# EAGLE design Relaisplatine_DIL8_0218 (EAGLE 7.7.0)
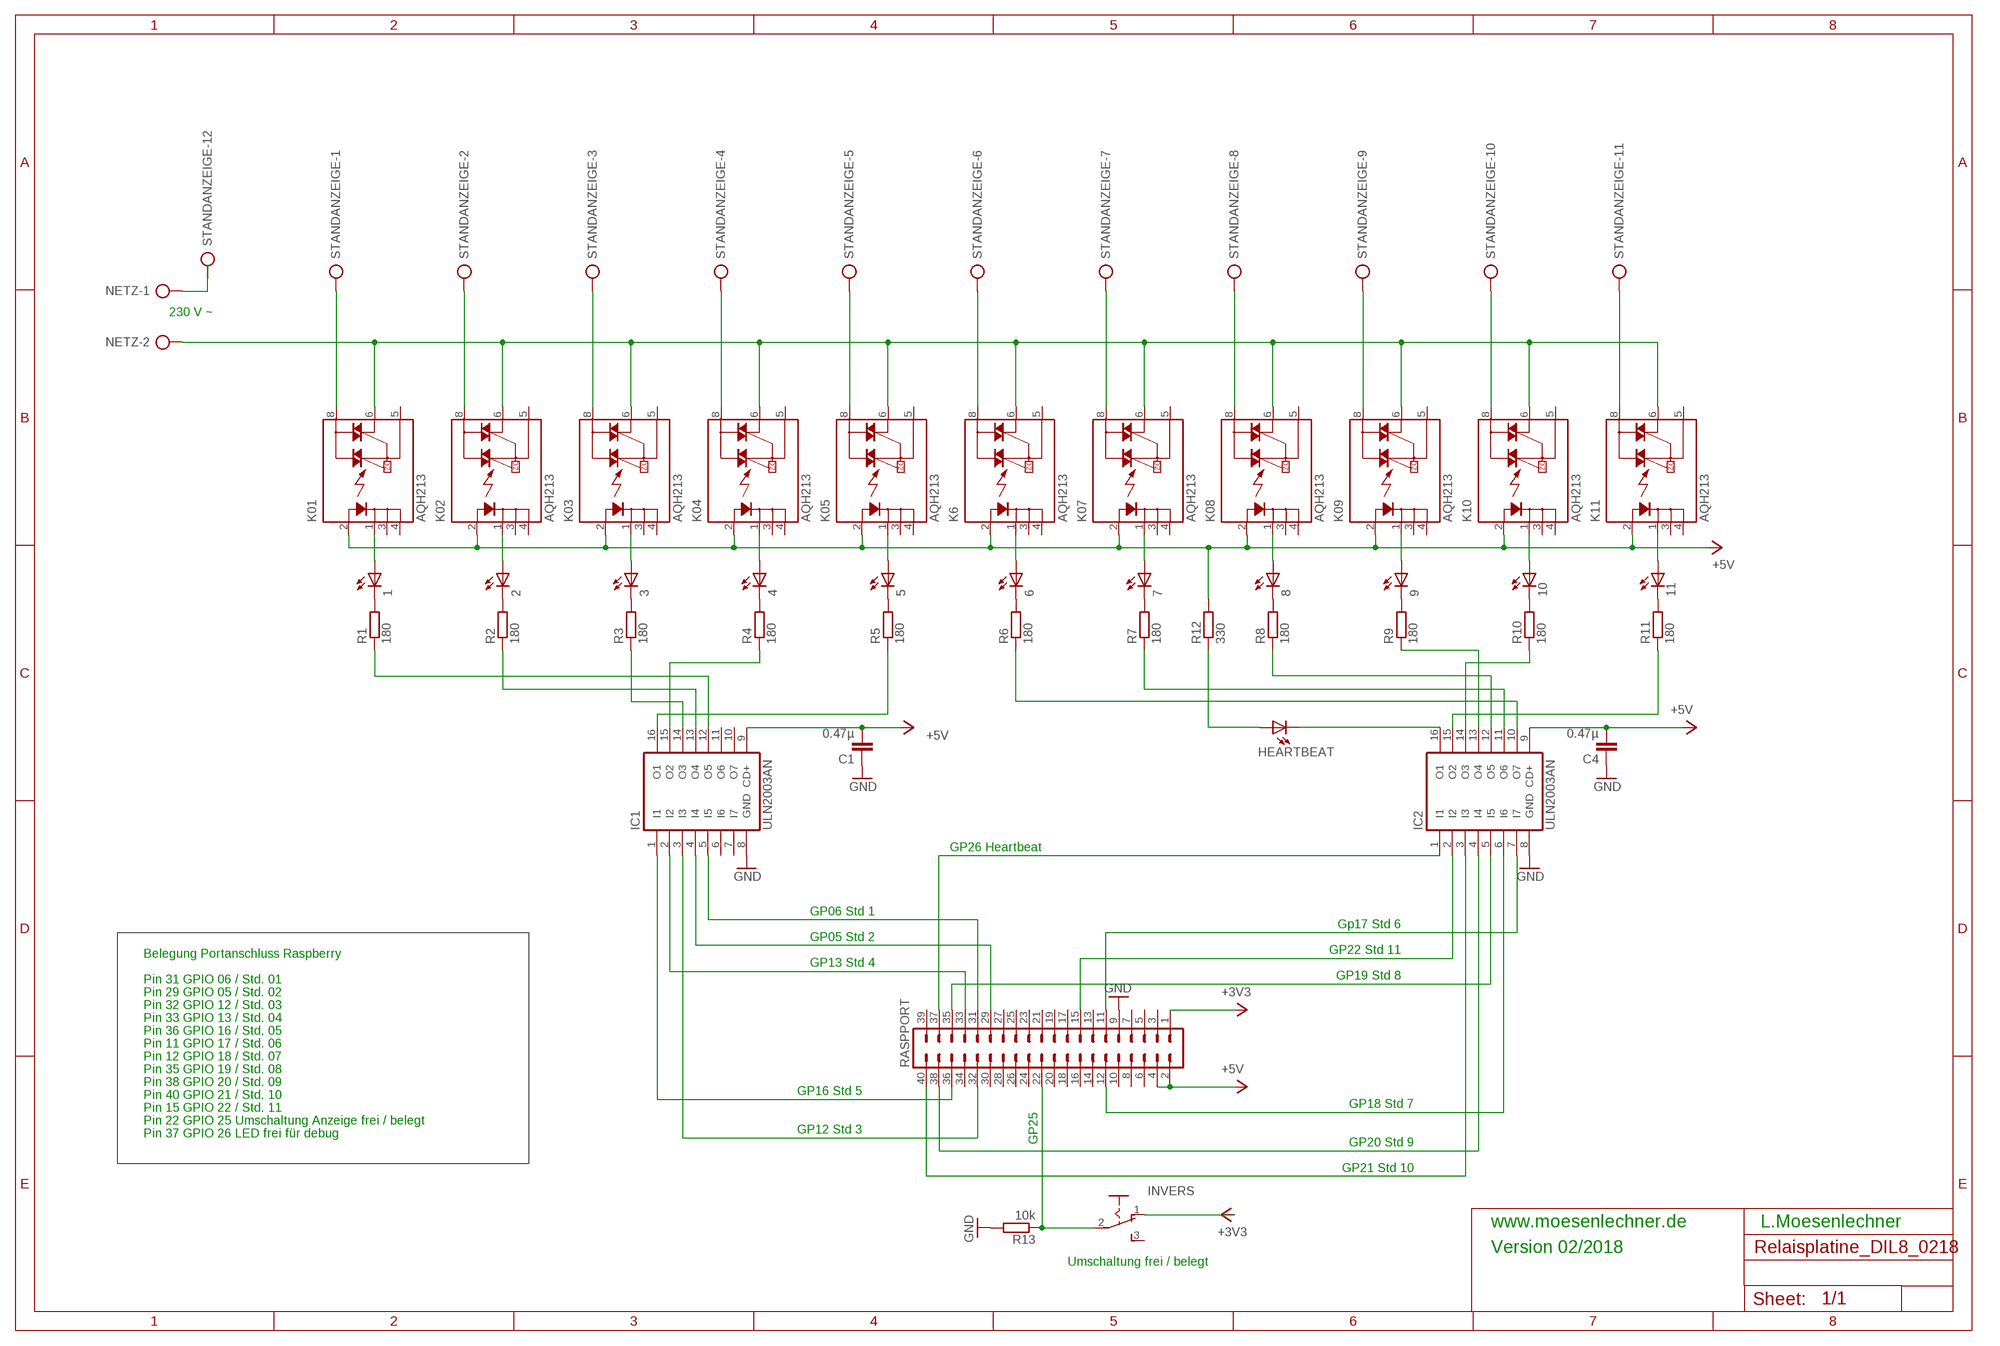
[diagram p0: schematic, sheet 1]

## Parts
1  LS_T679-D2E2-1  [PLCC2]
2  LS_T679-D2E2-1  [PLCC2]
3  LS_T679-D2E2-1  [PLCC2]
4  LS_T679-D2E2-1  [PLCC2]
5  LS_T679-D2E2-1  [PLCC2]
6  LS_T679-D2E2-1  [PLCC2]
7  LS_T679-D2E2-1  [PLCC2]
8  LS_T679-D2E2-1  [PLCC2]
9  LS_T679-D2E2-1  [PLCC2]
10  LS_T679-D2E2-1  [PLCC2]
11  LS_T679-D2E2-1  [PLCC2]
C1  0.47µ  C-EUC1206K  [C1206K]
C4  0.47µ  C-EUC1206K  [C1206K]
HEARTBEAT  LS_T679-D2E2-1  [PLCC2]
IC1  ULN2003AN  [DIL16]
IC2  ULN2003AN  [DIL16]
INVERS  M251  [M251]
K01  AQH213  [DIL07]
K02  AQH213  [DIL07]
K03  AQH213  [DIL07]
K04  AQH213  [DIL07]
K05  AQH213  [DIL07]
K6  AQH213  [DIL07]
K07  AQH213  [DIL07]
K08  AQH213  [DIL07]
K09  AQH213  [DIL07]
K10  AQH213  [DIL07]
K11  AQH213  [DIL07]
NETZ  AK500/2-H  [AK500/2-H]
R1  180  R-EU_R1206W  [R1206W]
R2  180  R-EU_R1206W  [R1206W]
R3  180  R-EU_R1206W  [R1206W]
R4  180  R-EU_R1206W  [R1206W]
R5  180  R-EU_R1206W  [R1206W]
R6  180  R-EU_R1206W  [R1206W]
R7  180  R-EU_R1206W  [R1206W]
R8  180  R-EU_R1206W  [R1206W]
R9  180  R-EU_R1206W  [R1206W]
R10  180  R-EU_R1206W  [R1206W]
R11  180  R-EU_R1206W  [R1206W]
R12  330  R-EU_R1206W  [R1206W]
R13  10k  R-EU_R1206W  [R1206W]
RASPPORT  MA20-2  [MA20-2]
STANDANZEIGE  AK500/12-H  [AK500/12-H]

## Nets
+3V3: INVERS.1(O) RASPPORT.1
+5V: C1.2 C4.2 IC1.9(CD+) IC2.9(CD+) K01.2(A) K02.2(A) K03.2(A) K04.2(A) K05.2(A) K6.2(A) K07.2(A) K08.2(A) K09.2(A) K10.2(A) K11.2(A) R12.2 RASPPORT.2 RASPPORT.4
GND: C1.1 C4.1 IC1.8(GND) IC2.8(GND) R13.2 RASPPORT.9
N$1: K01.8(DS1) STANDANZEIGE.1
N$2: K02.8(DS1) STANDANZEIGE.2
N$3: K03.8(DS1) STANDANZEIGE.3
N$4: K04.8(DS1) STANDANZEIGE.4
N$5: K05.8(DS1) STANDANZEIGE.5
N$6: K6.8(DS1) STANDANZEIGE.6
N$7: K07.8(DS1) STANDANZEIGE.7
N$8: K08.8(DS1) STANDANZEIGE.8
N$9: K09.8(DS1) STANDANZEIGE.9
N$10: K10.8(DS1) STANDANZEIGE.10
N$11: K11.8(DS1) STANDANZEIGE.11
N$12: K01.6(DS3) K02.6(DS3) K03.6(DS3) K04.6(DS3) K05.6(DS3) K6.6(DS3) K07.6(DS3) K08.6(DS3) K09.6(DS3) K10.6(DS3) K11.6(DS3) NETZ.2
N$13: 9.C R9.2
N$14: IC1.16(O1) R5.1
N$15: IC1.5(I5) RASPPORT.31
N$16: 10.C R10.2
N$17: 2.C R2.2
N$18: IC1.13(O4) R2.1
N$19: 11.C R11.2
N$20: IC2.10(O7) R6.1
N$21: IC2.11(O6) R7.1
N$22: 3.C R3.2
N$23: 4.C R4.2
N$24: 5.C R5.2
N$25: IC2.12(O5) R8.1
N$26: IC2.4(I4) RASPPORT.38
N$27: IC2.13(O4) R9.1
N$28: IC2.15(O2) R11.1
N$29: IC2.14(O3) R10.1
N$30: IC2.7(I7) RASPPORT.11
N$31: IC1.14(O3) R3.1
N$32: IC1.15(O2) R4.1
N$33: IC1.12(O5) R1.1
N$35: IC2.6(I6) RASPPORT.12
N$36: IC2.5(I5) RASPPORT.35
N$37: IC2.3(I3) RASPPORT.40
N$38: 1.C R1.2
N$39: 6.C R6.2
N$40: 7.C R7.2
N$41: 8.C R8.2
N$42: IC2.2(I2) RASPPORT.15
N$43: NETZ.1 STANDANZEIGE.12
N$44: 1.A K01.1(K)
N$45: 2.A K02.1(K)
N$46: 3.A K03.1(K)
N$47: 4.A K04.1(K)
N$48: 5.A K05.1(K)
N$49: 6.A K6.1(K)
N$50: IC1.1(I1) RASPPORT.36
N$51: IC1.3(I3) RASPPORT.32
N$52: IC1.2(I2) RASPPORT.33
N$53: 7.A K07.1(K)
N$54: 8.A K08.1(K)
N$55: 9.A K09.1(K)
N$56: 10.A K10.1(K)
N$57: 11.A K11.1(K)
N$58: HEARTBEAT.C IC2.16(O1)
N$59: HEARTBEAT.A R12.1
N$60: INVERS.2(P) R13.1 RASPPORT.22
N$61: IC2.1(I1) RASPPORT.37
N$62: IC1.4(I4) RASPPORT.29
Unconnected: IC1.6(I6) IC1.7(I7) IC1.10(O7) IC1.11(O6) INVERS.3(S) K01.3(K1) K01.4(K2) K01.5(DS2) K02.3(K1) K02.4(K2) K02.5(DS2) K03.3(K1) K03.4(K2) K03.5(DS2) K04.3(K1) K04.4(K2) K04.5(DS2) K05.3(K1) K05.4(K2) K05.5(DS2) K6.3(K1) K6.4(K2) K6.5(DS2) K07.3(K1) K07.4(K2) K07.5(DS2) K08.3(K1) K08.4(K2) K08.5(DS2) K09.3(K1) K09.4(K2) K09.5(DS2) K10.3(K1) K10.4(K2) K10.5(DS2) K11.3(K1) K11.4(K2) K11.5(DS2) RASPPORT.3 RASPPORT.5 RASPPORT.6 RASPPORT.7 RASPPORT.8 RASPPORT.10 RASPPORT.13 RASPPORT.14 RASPPORT.16 RASPPORT.17 RASPPORT.18 RASPPORT.19 RASPPORT.20 RASPPORT.21 RASPPORT.23 RASPPORT.24 RASPPORT.25 RASPPORT.26 RASPPORT.27 RASPPORT.28 RASPPORT.30 RASPPORT.34 RASPPORT.39

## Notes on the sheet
- 230 V ~
- GP26 Heartbeat
- GP06 Std 1
- Gp17 Std 6
- GP05 Std 2
- GP22 Std 11
- Belegung Portanschluss Raspberry | GP13 Std 4
- GP19 Std 8
- Pin 31 GPIO 06 / Std. 01
- Pin 29 GPIO 05 / Std. 02
- Pin 32 GPIO 12 / Std. 03
- Pin 33 GPIO 13 / Std. 04
- Pin 36 GPIO 16 / Std. 05
- Pin 11 GPIO 17 / Std. 06
- Pin 12 GPIO 18 / Std. 07
- Pin 35 GPIO 19 / Std. 08
- Pin 38 GPIO 20 / Std. 09 | GP16 Std 5
- Pin 40 GPIO 21 / Std. 10 | GP18 Std 7
- Pin 15 GPIO 22 / Std. 11 | GP25
- Pin 22 GPIO 25 Umschaltung Anzeige frei / belegt | GP12 Std 3
- Pin 37 GPIO 26 LED frei für debug | GP20 Std 9
- GP21 Std 10
- www.moesenlechner.de | L.Moesenlechner
- Version 02/2018
- Umschaltung frei / belegt

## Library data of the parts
1-11 HEARTBEAT = led:*_T679-?-1: LC TOPLED® Low Current LED; COLOR: super-red
C1 C4 = rcl:C-EU: CAPACITOR, European symbol
IC1 IC2 = uln-udn:ULN2003A: DRIVER ARRAY
INVERS = switch:M251: SLIDING SWITCH Mors, distributor Buerklin, 11G702
K01-K05 K6 K07-K09 K10 K11 = relay:AQH*213: SOLID STATE RELAY NAiS Source: http://www.mew-europe.com/.. en_ds_61613_0000.pdf; OC_FARNELL: unknown; OC_NEWARK: unknown
NETZ = con-ptr500:AK500/2-H: CONNECTOR; OC_FARNELL: unknown; OC_NEWARK: unknown
R1-R13 = rcl:R-EU_: RESISTOR, European symbol
RASPPORT = con-lstb:MA20-2: PIN HEADER; OC_FARNELL: unknown; OC_NEWARK: unknown
STANDANZEIGE = con-ptr500:AK500/12-H: CONNECTOR Aug. 2004 / PTR Meßtechnik: Die Bezeichnung der Serie AK505 wurde geändert. Es handelt sich hierbei um AK500 in horizontaler Ausführung.; OC_FARNELL: unknown; OC_NEWARK: unknown

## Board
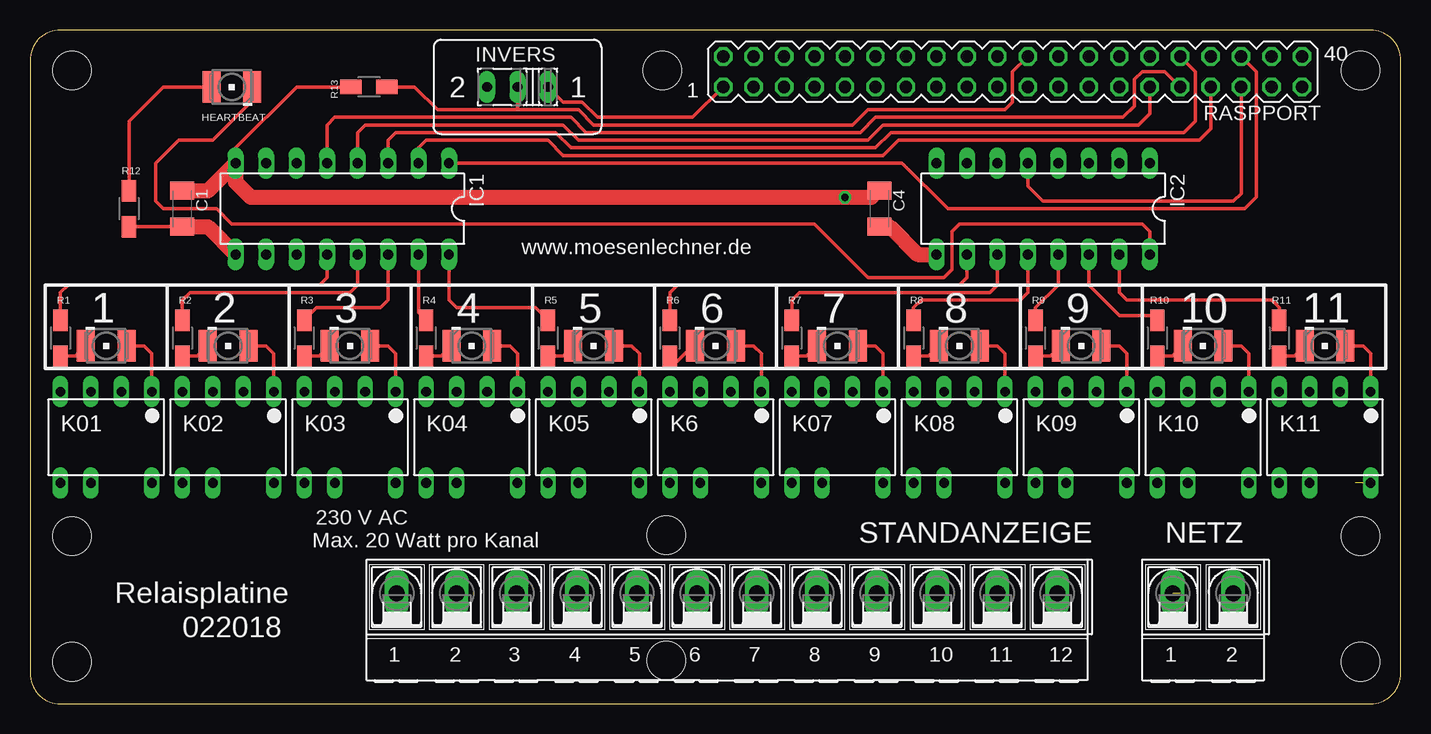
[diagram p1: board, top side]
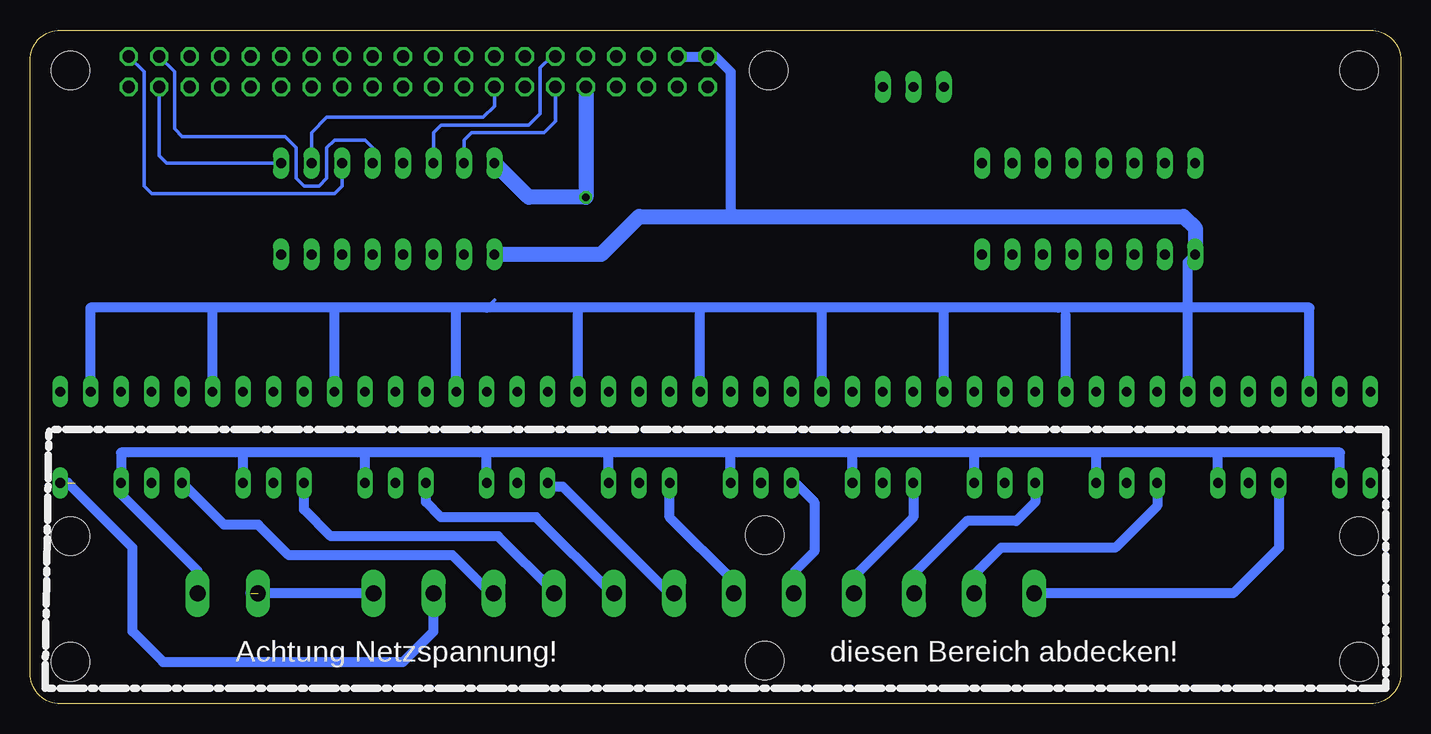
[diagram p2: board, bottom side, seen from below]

Size 114.28 x 56.19 mm. Coordinates in mm from the lower left corner, seen from the top.
Outline: 0,53.65 0,2.54 arc90 2.54,0 111.74,0 arc90 114.28,2.54 114.28,53.65 arc90 111.74,56.19 2.54,56.19 arc90 0,53.65
Copper layers (1*16): Top 0.035mm / dielectric 1.5mm / Bottom 0.035mm
Design rules "default": minimum track width 10mil, minimum drill 24mil, track to track 8mil, track to pad 8mil, pad to pad 8mil, via to via 8mil, smd to smd 8mil, copper to edge 40mil, drill to drill 8mil, minimum pad ring 10mil, minimum via ring 8mil, stop-mask expansion 4mil, vias tented up to drill 0mil, thermal gap 10mil
Holes 3.2 mm at 3.5,52.8 110.92,52.8 110.92,3.5 3.5,3.5 52.71,52.8 53.03,3.59 110.92,13.98 3.5,13.98 53.03,14.06

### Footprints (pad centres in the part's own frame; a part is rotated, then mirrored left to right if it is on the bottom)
PLCC2 = smd 2.6 x 1.5: A 0,1.7; C 0,-1.7
C1206K = smd 1.5 x 2: 1 -1.5,0; 2 1.5,0
DIL16 = drill 0.813 long: 1 -8.89,-3.81; 2 -6.35,-3.81; 3 -3.81,-3.81; 4 -1.27,-3.81; 5 1.27,-3.81; 6 3.81,-3.81; 7 6.35,-3.81; 8 8.89,-3.81; 9 8.89,3.81; 10 6.35,3.81; 11 3.81,3.81; 12 1.27,3.81; 13 -1.27,3.81; 14 -3.81,3.81; 15 -6.35,3.81; 16 -8.89,3.81
M251 = drill 0.813 long: 1 -2.54,0; 2 0,0; 3 2.54,0
DIL07 = drill 0.8 long: 1 -3.81,-3.81; 2 -1.27,-3.81; 3 1.27,-3.81; 4 3.81,-3.81; 5 3.81,3.81; 6 1.27,3.81; 8 -3.81,3.81
AK500/2-H = drill 1.321 long: 1 -2.515,0; 2 2.515,0
R1206W = smd 1.8 x 1.2: 1 -1.499,0; 2 1.499,0
MA20-2 = drill 1.016 octagon: 1 -24.13,-1.27; 2 -24.13,1.27; 3 -21.59,-1.27; 4 -21.59,1.27; 5 -19.05,-1.27; 6 -19.05,1.27; 7 -16.51,-1.27; 8 -16.51,1.27; 9 -13.97,-1.27; 10 -13.97,1.27; 11 -11.43,-1.27; 12 -11.43,1.27; 13 -8.89,-1.27; 14 -8.89,1.27; 15 -6.35,-1.27; 16 -6.35,1.27; 17 -3.81,-1.27; 18 -3.81,1.27; 19 -1.27,-1.27; 20 -1.27,1.27; 21 1.27,-1.27; 22 1.27,1.27; 23 3.81,-1.27; 24 3.81,1.27; 25 6.35,-1.27; 26 6.35,1.27; 27 8.89,-1.27; 28 8.89,1.27; 29 11.43,-1.27; 30 11.43,1.27; 31 13.97,-1.27; 32 13.97,1.27; 33 16.51,-1.27; 34 16.51,1.27; 35 19.05,-1.27; 36 19.05,1.27; 37 21.59,-1.27; 38 21.59,1.27; 39 24.13,-1.27; 40 24.13,1.27
AK500/12-H = drill 1.321 long: 1 -27.534,0; 2 -22.53,0; 3 -17.526,0; 4 -12.497,0; 5 -7.493,0; 6 -2.489,0; 7 2.489,0; 8 7.493,0; 9 12.497,0; 10 17.526,0; 11 22.53,0; 12 27.534,0

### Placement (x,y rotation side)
1  6.35,29.84 270 top
2  16.51,29.84 270 top
3  26.67,29.84 270 top
4  36.83,29.84 270 top
5  46.99,29.84 270 top
6  57.15,29.84 270 top
7  67.31,29.84 270 top
8  77.47,29.84 270 top
9  87.63,29.84 270 top
10  97.79,29.84 270 top
11  107.95,29.84 270 top
C1  12.7,41.27 270 top
C4  70.8,41.27 270 top
HEARTBEAT  16.83,51.44 90 top
IC1  26.04,41.27 180 top
IC2  84.45,41.27 180 top
INVERS  40.64,51.44 180 top
K01  6.35,22.23 180 top
K02  16.51,22.23 180 top
K03  26.67,22.23 180 top
K04  36.83,22.23 180 top
K05  46.99,22.23 180 top
K6  57.15,22.23 180 top
K07  67.31,22.23 180 top
K08  77.47,22.23 180 top
K09  87.63,22.23 180 top
K10  97.79,22.23 180 top
K11  107.95,22.23 180 top
NETZ  97.79,9.21 0 top
R1  2.54,30.48 270 top
R2  12.7,30.48 270 top
R3  22.86,30.48 270 top
R4  33.02,30.48 270 top
R5  43.18,30.48 270 top
R6  53.34,30.48 270 top
R7  63.5,30.48 270 top
R8  73.66,30.48 270 top
R9  83.82,30.48 270 top
R10  93.98,30.48 270 top
R11  104.14,30.48 270 top
R12  8.26,41.27 270 top
R13  28.26,51.44 180 top
RASPPORT  81.92,52.7 0 top
STANDANZEIGE  58.1,9.21 0 top

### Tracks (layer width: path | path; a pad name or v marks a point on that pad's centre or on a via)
+3V3
  Top 0.305: INVERS.1 44.45,50.16 46.04,50.16 47.31,48.9 55.24,48.9 RASPPORT.1
+5V
  Top 0.305: C1.2 R12.2 | 71.67,39.77 C4.2 70.72,39.77 | 70.72,39.77 70.48,40.01 | 70.8,39.69 70.72,39.77
  Top 1.27: C1.2 14.84,39.77 IC1.9 | 71.67,39.77 73.98,37.47 IC2.9
  Bottom 0.305: 27.94,32.38 28.57,33.02 | 75.56,33.66 76.2,33.02 | RASPPORT.2 RASPPORT.4
  Bottom 0.813: 58.42,33.02 68.58,33.02 | 68.58,33.02 76.2,33.02 78.74,33.02 | 78.74,33.02 88.9,33.02 | 88.9,33.02 99.06,33.02 | 99.06,33.02 109.22,33.02 K11.2 | K01.2 7.62,33.02 17.78,33.02 | 17.78,33.02 28.57,33.02 38.1,33.02 | 38.1,33.02 48.26,33.02 | 48.26,33.02 58.42,33.02 | K02.2 17.78,33.02 | K03.2 27.94,32.38 | K04.2 38.1,33.02 | K05.2 48.26,33.02 | K6.2 58.42,33.02 | K07.2 68.58,33.02 | K08.2 78.74,33.02 | K09.2 88.9,33.02 | K10.2 99.06,33.02 | 17.78,33.02 17.78,36.83 IC1.9 | RASPPORT.4 57.15,53.98 55.88,52.7 55.88,40.96 55.56,40.64
  Bottom 1.27: IC1.9 17.14,39.69 18.1,40.64 55.56,40.64 63.5,40.64 66.67,37.47 IC2.9
GND  (via drill 0.6)
  Top 0.305: IC1.8 17.14,46.35 22.23,51.44 R13.2
  Top 0.406: 70.17,42.23 70.8,42.23 C4.1
  Top 1.27: 70.17,42.23 v67.94,42.23 18.41,42.23 17.14,43.5 IC1.8 14.84,42.77 C1.1
  Bottom 1.27: IC2.8 72.71,42.23 v67.94,42.23 RASPPORT.9
N$1
  Bottom 0.813: K01.8 10.16,13.02 13.97,9.21 STANDANZEIGE.1
N$2
  Bottom 0.813: K02.8 20.32,16.51 23.81,13.02 33.34,13.02 35.56,10.79 STANDANZEIGE.2
N$3
  Bottom 0.813: K03.8 30.48,16.83 32.07,15.24 36.2,15.24 40.64,10.79 40.64,9.27 STANDANZEIGE.3
N$4
  Bottom 0.813: K04.8 40.64,15.56 45.4,10.79 45.4,9.41 STANDANZEIGE.4
N$5
  Bottom 0.813: K05.8 50.48,18.41 48.9,16.83 48.9,12.7 50.48,11.11 50.48,9.34 STANDANZEIGE.5
N$6
  Bottom 0.813: STANDANZEIGE.6 55.61,10.21 60.96,15.56 K6.8
N$7
  Bottom 0.813: STANDANZEIGE.7 60.96,9.21 69.85,18.1 70.8,18.1 K07.8
N$8
  Bottom 0.813: STANDANZEIGE.8 65.72,9.21 72.07,15.56 80.01,15.56 81.28,16.83 K08.8
N$9
  Bottom 0.813: STANDANZEIGE.9 70.6,9.32 75.25,13.97 89.22,13.97 91.44,16.19 K09.8
N$10
  Bottom 0.813: STANDANZEIGE.10 75.88,9.21 79.06,12.38 92.71,12.38 95.25,14.92 98.11,14.92 K10.8
N$11  (1 unrouted)
  Bottom 0.813: K11.8 111.12,18.41 105.73,13.02 105.73,6.03 103.19,3.49 83.19,3.49 80.64,6.03 80.64,9.2 STANDANZEIGE.11
N$12
  Bottom 0.813: K01.6 5.08,20.95 15.24,20.95 | 15.24,20.95 25.4,20.95 | 25.4,20.95 35.56,20.95 | 35.56,20.95 45.72,20.95 | 45.72,20.95 55.88,20.95 | 55.88,20.95 66.04,20.95 | 66.04,20.95 76.2,20.95 | 76.2,20.95 86.36,20.95 | 86.36,20.95 96.52,20.95 | 96.52,20.95 106.68,20.95 K11.6 106.68,17.46 100.31,11.09 NETZ.2 | K02.6 15.24,20.95 | K03.6 25.4,20.95 | K04.6 35.56,20.95 | K05.6 45.72,20.95 | K6.6 55.88,20.95 | K07.6 66.04,20.95 | K08.6 76.2,20.95 | K09.6 86.36,20.95 | K10.6 96.52,20.95
N$13
  Top 0.305: R9.2 85.07,28.98 9.C
N$14
  Top 0.305: IC1.16 34.92,33.66 35.56,33.02 42.14,33.02 R5.1
N$15
  Top 0.305: IC1.5 24.77,48.26 25.4,48.9 45.09,48.9 46.35,47.62 69.22,47.62 70.48,48.9 91.12,48.9 92.08,49.85 92.08,52.07 92.71,52.7 94.61,52.7 RASPPORT.31
N$16
  Top 0.305: R10.2 95.23,28.98 10.C
N$17
  Top 0.305: R2.2 13.95,28.98 2.C
N$18
  Top 0.305: IC1.13 27.3,34.92 26.67,34.29 13.34,34.29 12.7,33.66 R2.1
N$19
  Top 0.305: R11.2 105.39,28.98 11.C
N$20
  Top 0.305: IC2.10 78.11,35.56 77.47,34.92 53.98,34.92 53.34,34.29 R6.1
N$21
  Top 0.305: IC2.11 80.64,34.92 80.01,34.29 64.14,34.29 63.5,33.66 R7.1
N$22
  Top 0.305: R3.2 24.11,28.98 3.C
N$23
  Top 0.305: R4.2 34.27,28.98 4.C
N$24
  Top 0.305: R5.2 44.43,28.98 5.C
N$25
  Top 0.305: IC2.12 83.19,34.29 82.55,33.66 74.3,33.66 73.66,33.02 R8.1
N$26
  Bottom 0.305: IC2.4 85.72,46.35 86.36,46.99 88.9,46.99 89.53,46.35 89.53,43.81 90.17,43.18 91.44,43.18 92.08,43.81 92.08,46.35 93.03,47.31 101.6,47.31 102.23,47.94 102.23,52.7 RASPPORT.38
N$27
  Top 0.305: IC2.13 85.72,34.92 83.82,33.02 R9.1
N$28
  Top 0.305: IC2.15 90.81,34.29 91.44,33.66 103.5,33.66 104.14,33.02 R11.1
N$29
  Top 0.305: IC2.14 88.27,34.92 90.81,32.38 93.57,32.38 R10.1
N$30
  Bottom 0.305: IC2.7 78.11,46.99 77.47,47.62 71.44,47.62 70.48,48.58 RASPPORT.11
N$31
  Top 0.305: IC1.14 29.84,33.66 29.21,33.02 23.9,33.02 R3.1
N$32
  Top 0.305: IC1.15 32.38,32.61 R4.1
N$33
  Top 0.305: IC1.12 24.77,35.56 24.13,34.92 3.17,34.92 2.54,34.29 R1.1
N$35
  Bottom 0.305: IC2.6 80.64,47.62 80.01,48.26 72.71,48.26 71.75,49.21 71.75,53.02 70.8,53.98 RASPPORT.12
N$36
  Top 0.305: IC2.5 83.19,43.18 84.45,41.91 100.33,41.91 100.97,42.55 RASPPORT.35
N$37
  Bottom 0.305: RASPPORT.40 104.78,52.7 104.78,43.18 104.14,42.55 88.9,42.55 88.27,43.18 IC2.3
N$38
  Top 0.305: R1.2 3.79,28.98 1.C
N$39
  Top 0.305: 6.C 55.24,29.84 53.98,28.57 53.75,28.57 R6.2
N$40
  Top 0.305: R7.2 64.75,28.98 7.C
N$41
  Top 0.305: R8.2 74.91,28.98 8.C
N$42
  Bottom 0.305: IC2.2 90.81,47.62 89.53,48.9 76.52,48.9 75.56,49.85 RASPPORT.15
N$43  (1 unrouted)
  Bottom 0.813: STANDANZEIGE.12 95.89,9.21
N$44
  Top 0.305: K01.1 10.16,29.21 9.53,29.84 1.A
N$45
  Top 0.305: K02.1 20.32,29.21 19.68,29.84 2.A
N$46
  Top 0.305: K03.1 30.48,29.21 29.84,29.84 3.A
N$47
  Top 0.305: K04.1 40.64,29.21 40.01,29.84 4.A
N$48
  Top 0.305: K05.1 50.8,29.21 50.16,29.84 5.A
N$49
  Top 0.305: K6.1 60.96,29.21 60.33,29.84 6.A
N$50
  Top 0.305: RASPPORT.36 102.23,52.7 102.23,42.23 101.28,41.27 76.52,41.27 72.71,45.09 IC1.1
N$51
  Top 0.305: IC1.3 29.84,46.99 30.48,47.62 43.81,47.62 45.09,46.35 70.48,46.35 71.75,47.62 96.2,47.62 97.16,48.58 97.16,52.7 RASPPORT.32
N$52
  Top 0.305: IC1.2 32.38,46.35 33.02,46.99 43.18,46.99 44.45,45.72 71.12,45.72 72.39,46.99 97.47,46.99 98.42,47.94 RASPPORT.33
N$53
  Top 0.305: K07.1 71.12,29.21 70.48,29.84 7.A
N$54
  Top 0.305: K08.1 81.28,29.21 80.64,29.84 8.A
N$55
  Top 0.305: K09.1 91.44,29.21 90.81,29.84 9.A
N$56
  Top 0.305: K10.1 101.6,29.21 100.97,29.84 10.A
N$57
  Top 0.305: K11.1 111.76,29.21 111.12,29.84 11.A
N$58
  Top 0.305: IC2.16 93.34,39.37 92.71,40.01 77.47,40.01 76.83,39.37 76.83,36.2 76.2,35.56 69.85,35.56 65.41,40.01 16.83,40.01 15.56,41.27 11.11,41.27 10.48,41.91 10.48,45.09 12.38,46.99 15.24,46.99 18.73,50.48 18.73,51.23 HEARTBEAT.C 18.41,52.59
N$59
  Top 0.305: R12.1 8.26,48.58 11.11,51.44 HEARTBEAT.A
N$60
  Top 0.305: 40.64,49.53 33.97,49.53 32.07,51.44 R13.1 | RASPPORT.22 81.92,52.7 81.92,50.16 81.28,49.53 69.85,49.53 68.58,48.26 46.99,48.26 45.72,49.53 40.64,49.53 | INVERS.2 40.64,49.53
N$61
  Bottom 0.305: IC2.1 102.87,45.09 103.5,45.72 RASPPORT.37
N$62
  Top 0.305: IC1.4 27.3,47.62 27.94,48.26 44.45,48.26 45.72,46.99 69.85,46.99 71.12,48.26 92.39,48.26 93.34,49.21 RASPPORT.29

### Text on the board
bPlace: diesen Bereich abdecken! | Achtung Netzspannung!
tNames: www.moesenlechner.de | 230 V AC | Max. 20 Watt pro Kanal | Relaisplatine | 022018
